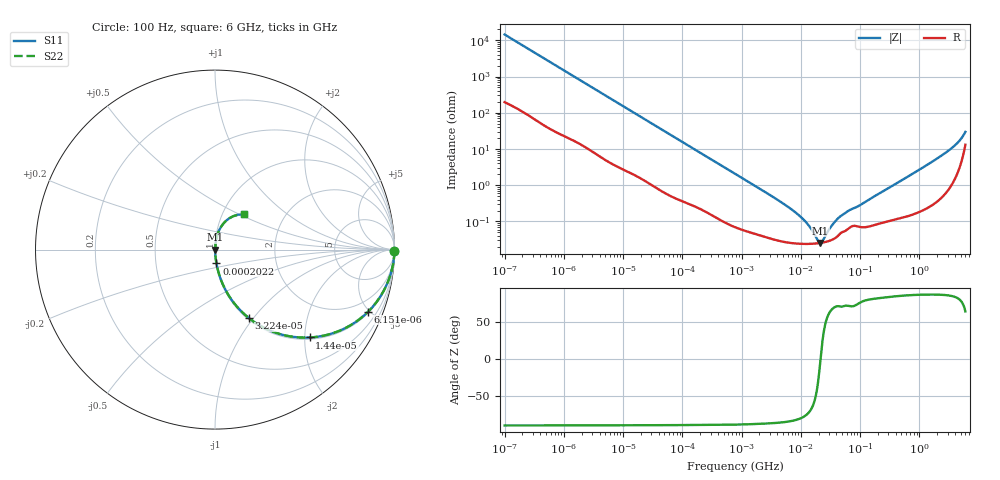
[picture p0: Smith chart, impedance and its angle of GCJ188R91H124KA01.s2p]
!Murata Part Number: GCJ188R91H124KA01
!These Parameters are Measured in Series Mode Connection
!Data Generated on Mar 13, 2026
!  o--ll--o
!Port1  Port2
!  o------o
!Operation Temp=25[degC], DC Bias Voltage=0[V]
!Freq. Start=100[Hz] Stop=6[GHz] 401[Steps]
# Hz S RI R 50
!Freq.(Hz) S11(Real) S11(Imag) S21(Real) S21(Imag) S12(Real) S12(Imag) S22(Real) S22(Imag)
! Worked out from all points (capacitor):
!   401 points, 100 Hz to 6 GHz, reference 50 ohm
!   read as one part in series: C = 110 nF near 109 Hz
!   lowest |Z| = 25.6 mohm at 21.28 MHz (marker M1)
!   series resonance near 21.54 MHz, so ESL is about 500 pH
!   S11 on the Smith chart (normalised r, x): 100 Hz: open; 6.151 kHz: 1.08, -4.90; 14.4 kHz: 1.04, -2.11; 32.24 kHz: 1.02, -0.95; 202.2 kHz: 1.00, -0.16; 6 GHz: 1.26, +0.53
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100  0.9999 -0.0069  0.000141 0.0069  0.000141 0.0069  0.9999 -0.0069
600  0.9978 -0.0406  0.00223 0.0406  0.00223 0.0406  0.9978 -0.0406
2008  0.98 -0.1317  0.02 0.1317  0.02 0.1317  0.98 -0.1317
6151  0.8533 -0.3456  0.1467 0.3456  0.1467 0.3456  0.8533 -0.3456
14402  0.527 -0.4897  0.473 0.4897  0.473 0.4897  0.527 -0.4897
32244  0.1903 -0.3827  0.8097 0.3827  0.8097 0.3827  0.1903 -0.3827
40335  0.1325 -0.3293  0.8675 0.3293  0.8675 0.3293  0.1325 -0.3293
75495  0.0444 -0.1956  0.9556 0.1956  0.9556 0.1956  0.0444 -0.1956
202169  0.00819 -0.0771  0.9918 0.0771  0.9918 0.0771  0.00819 -0.0771
774597  0.00112 -0.0207  0.9989 0.0207  0.9989 0.0207  0.00112 -0.0207
6644369  0.000261 -0.00227  0.9997 0.00227  0.9997 0.00227  0.000261 -0.00227
1.087309e7  0.000242 -0.00115  0.9998 0.00115  0.9998 0.00115  0.000242 -0.00115
1.555665e7  0.000243 -0.000515  0.9998 0.000515  0.9998 0.000515  0.000243 -0.000515
1.946e7  0.00025 -0.000158  0.9997 0.000158  0.9997 0.000158  0.00025 -0.000158
2.128304e7  0.000255 -1.85e-05  0.9997 1.85e-05  0.9997 1.85e-05  0.000255 -1.85e-05
2.327686e7  0.000261 0.000121  0.9997 -0.000121  0.9997 -0.000121  0.000261 0.000121
3.330331e7  0.00031 0.000705  0.9997 -0.000705  0.9997 -0.000705  0.00031 0.000705
4.556224e7  0.000453 0.00128  0.9995 -0.00128  0.9995 -0.00128  0.000453 0.00128
3.124326e8  0.0011 0.00856  0.9989 -0.00856  0.9989 -0.00856  0.0011 0.00856
2.562649e9  0.0101 0.0705  0.9899 -0.0705  0.9899 -0.0705  0.0101 0.0705
4.385646e9  0.0398 0.136  0.9602 -0.136  0.9602 -0.136  0.0398 0.136
6e9  0.1621 0.1967  0.8379 -0.1967  0.8379 -0.1967  0.1621 0.1967
